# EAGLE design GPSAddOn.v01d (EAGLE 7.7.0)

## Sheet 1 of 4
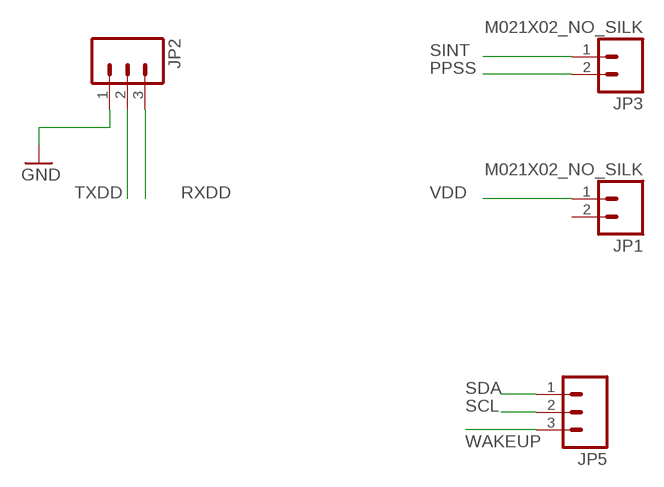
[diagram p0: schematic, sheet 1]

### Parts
JP1  M021X02_NO_SILK  [1X02_NO_SILK]
JP2  M031X03_NO_SILK  [1X03_NO_SILK]
JP3  M021X02_NO_SILK  [1X02_NO_SILK]
JP5  M031X03_NO_SILK  [1X03_NO_SILK]

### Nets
GND: JP2.1 ; also sheet 2,3,4
PPSS: JP3.2 ; also sheet 2
RXDD: JP2.3 ; also sheet 2
SCL: JP5.2 ; also sheet 2,4
SDA: JP5.1 ; also sheet 2,4
SINT: JP3.1 ; also sheet 4
TXDD: JP2.2 ; also sheet 2
VDD: JP1.1 ; also sheet 2,3,4
WAKEUP: JP5.3 ; also sheet 2
Unconnected: JP1.2

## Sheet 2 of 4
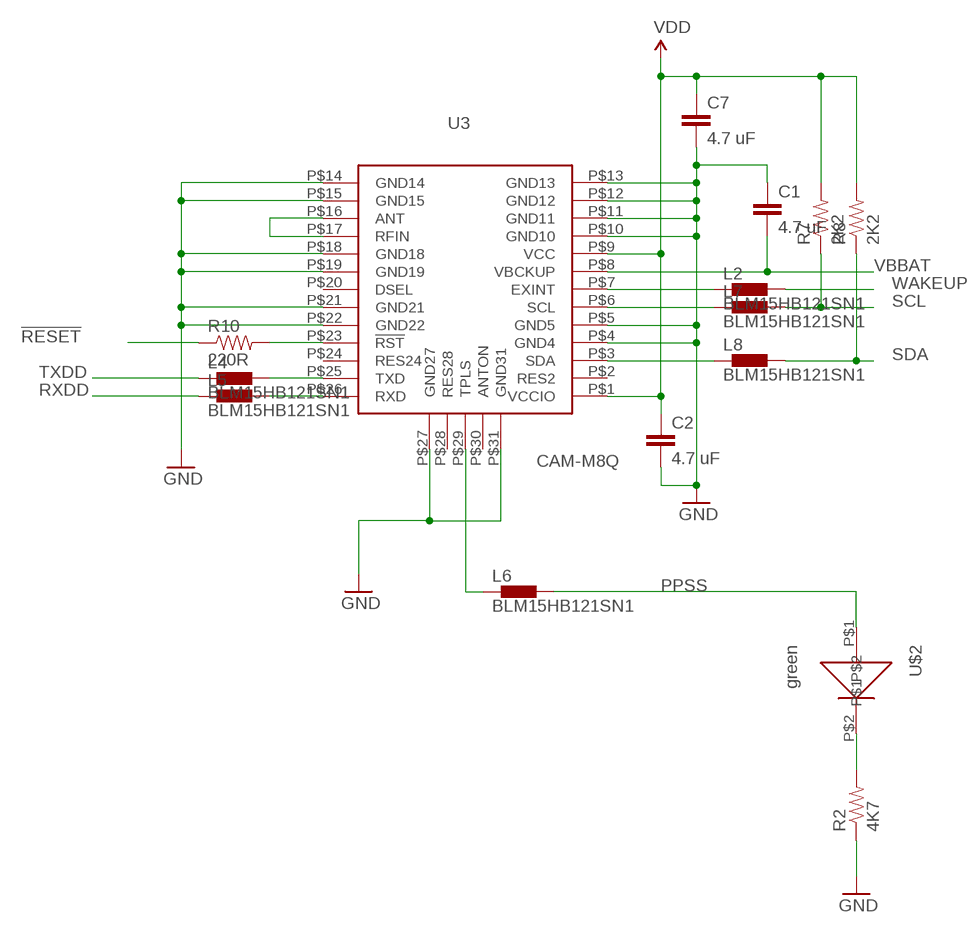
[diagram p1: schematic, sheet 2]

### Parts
C1  4.7 uF  0402CAP.KW  [0402-CAP]
C2  4.7 uF  0402CAP.KW  [0402-CAP]
C7  4.7 uF  0402CAP.KW  [0402-CAP]
L2  BLM15HB121SN1  [0402]
L4  BLM15HB121SN1  [0402]
L5  BLM15HB121SN1  [0402]
L6  BLM15HB121SN1  [0402]
L7  BLM15HB121SN1  [0402]
L8  BLM15HB121SN1  [0402]
R2  4K7  0402RES.KW  [0402-RES]
R7  2K2  0402RES.KW  [0402-RES]
R8  2K2  0402RES.KW  [0402-RES]
R10  220R  0402RES.KW  [0402-RES]
U3  CAM-M8Q  [CAM-M8Q]
U$2  green  0402LED  [0402LED]

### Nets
!RESET: R10.1
GND: C1.1 C2.2 C7.2 R2.1 U3.P$4(GND4) U3.P$5(GND5) U3.P$10(GND10) U3.P$11(GND11) U3.P$12(GND12) U3.P$13(GND13) U3.P$14(GND14) U3.P$15(GND15) U3.P$18(GND18) U3.P$19(GND19) U3.P$21(GND21) U3.P$22(GND22) U3.P$27(GND27) U3.P$31(GND31) ; also sheet 1,3,4
N$6: L2.1 U3.P$7(EXINT)
N$10: L7.1 U3.P$6(SCL)
N$17: R2.2 U$2.P$2
N$23: L8.1 U3.P$3(SDA)
N$43: L4.2 U3.P$25(TXD)
N$44: L5.2 U3.P$26(RXD)
N$45: U3.P$16(ANT) U3.P$17(RFIN)
N$46: R10.2 U3.P$23(!RST)
N$47: L6.1 U3.P$29(TPLS)
PPSS: L6.2 U$2.P$1 ; also sheet 1
RXDD: L5.1 ; also sheet 1
SCL: L7.2 R7.1 ; also sheet 1,4
SDA: L8.2 R8.1 ; also sheet 1,4
TXDD: L4.1 ; also sheet 1
VBBAT: C1.2 U3.P$8(VBCKUP) ; also sheet 3
VDD: C2.1 C7.1 R7.2 R8.2 U3.P$1(VCCIO) U3.P$9(VCC) ; also sheet 1,3,4
WAKEUP: L2.2 ; also sheet 1
Unconnected: U3.P$2(RES2) U3.P$20(DSEL) U3.P$24(RES24) U3.P$28(RES28) U3.P$30(ANTON)

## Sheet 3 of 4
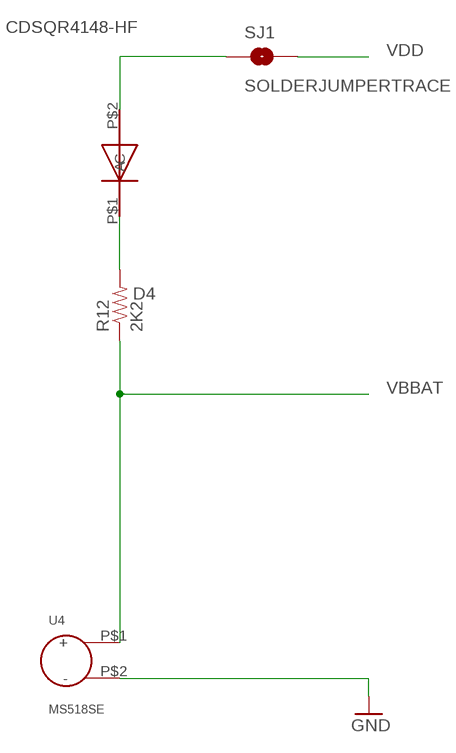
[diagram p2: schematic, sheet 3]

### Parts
D4  CDSQR4148-HF  [CDSQR4148-HF]
R12  2K2  0402RES.KW  [0402-RES]
SJ1  SOLDERJUMPERTRACE  [SJ_2S-TRACE]
U4  MS518SE  [MS518SE]

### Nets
GND: U4.P$2(-) ; also sheet 1,2,4
N$1: D4.P$1(C) R12.2
N$4: D4.P$2(A) SJ1.1
VBBAT: R12.1 U4.P$1(+) ; also sheet 2
VDD: SJ1.2 ; also sheet 1,2,4

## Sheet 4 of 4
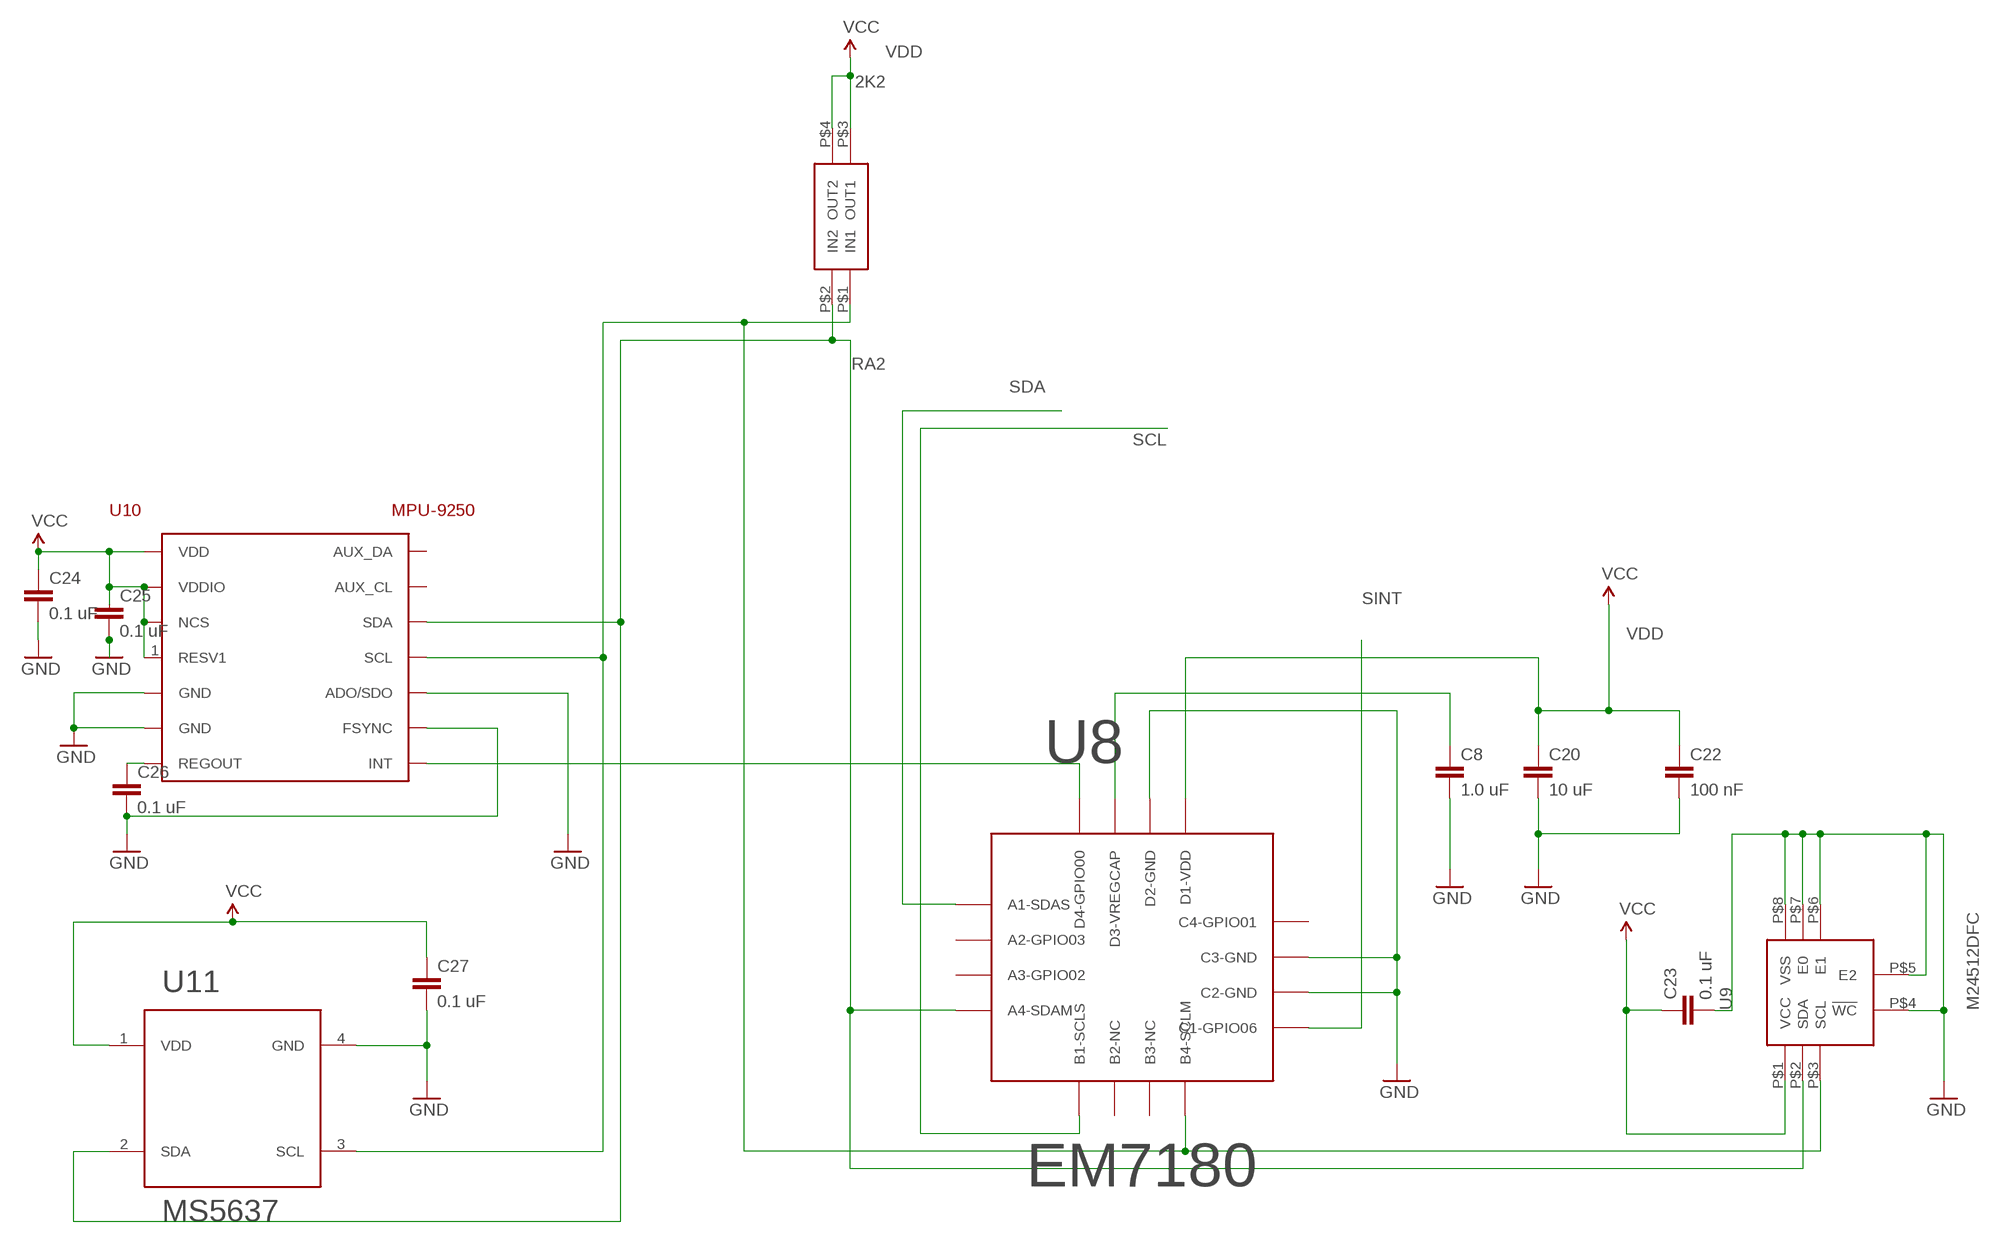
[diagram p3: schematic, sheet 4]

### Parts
C8  1.0 uF  CAP0402-CAP  [0402-CAP]
C20  10 uF  CAP0402-CAP  [0402-CAP]
C22  100 nF  CAP0402-CAP  [0402-CAP]
C23  0.1 uF  CAP0402-CAP  [0402-CAP]
C24  0.1 uF  CAP0402-CAP  [0402-CAP]
C25  0.1 uF  CAP0402-CAP  [0402-CAP]
C26  0.1 uF  CAP0402-CAP  [0402-CAP]
C27  0.1 uF  CAP0402-CAP  [0402-CAP]
RA2  2K2  EXB24V  [EXB24V]
U8  EM7180  [WL-CSP16]
U9  M24512DFC  [M24512DFC]
U10  MPU-9250  [MPU-9250]
U11  MS5637  [MS5637QFN-4]

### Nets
GND: C8.2 C20.2 C22.2 C23.2 C24.2 C25.2 C26.2 C27.2 U8.P$10(C2-GND) U8.P$11(C3-GND) U8.P$14(D2-GND) U9.P$4(!WC) U9.P$5(E2) U9.P$6(E1) U9.P$7(E0) U9.P$8(VSS) U10.9(ADO/SDO) U10.11(FSYNC) U10.18(GND) U10.20(GND) U11.4(GND) ; also sheet 1,2,3
N$19: U8.P$16(D4-GPIO00) U10.12(INT)
N$26: C8.1 U8.P$15(D3-VREGCAP)
N$40: C26.1 U10.10(REGOUT)
SCL: U8.P$5(B1-SCLS) ; also sheet 1,2
SCL2: RA2.P$1(IN1) U8.P$8(B4-SCLM) U9.P$3(SCL) U10.23(SCL) U11.3(SCL)
SDA: U8.P$1(A1-SDAS) ; also sheet 1,2
SDA2: RA2.P$2(IN2) U8.P$4(A4-SDAM) U9.P$2(SDA) U10.24(SDA) U11.2(SDA)
SINT: U8.P$9(C1-GPIO06) ; also sheet 1
VDD: C20.1 C22.1 C23.1 C24.1 C25.1 C27.1 RA2.P$3(OUT1) RA2.P$4(OUT2) U8.P$13(D1-VDD) U9.P$1(VCC) U10.1(RESV1) U10.8(VDDIO) U10.13(VDD) U10.22(NCS) U11.1(VDD) ; supply symbol labelled VCC ; also sheet 1,2,3
Unconnected: U8.P$2(A2-GPIO03) U8.P$3(A3-GPIO02) U8.P$6(B2-NC) U8.P$7(B3-NC) U8.P$12(C4-GPIO01) U10.7(AUX_CL) U10.21(AUX_DA)

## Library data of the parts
C1 C2 C7 = SparkFun-Capacitors:0402CAP.KW
C8 C20 C22-C27 = SparkFun-Capacitors:CAP: Capacitor
D4 = Kris:CDSQR4148-HF: ComChip's CDSQR4148-HF high speed 150 mA Io diode
JP1 JP3 = SparkFun-Connectors:M02: Standard 2-pin 0.1" header. Use with
JP2 JP5 = SparkFun-Connectors:M03: Header 3 Standard 3-pin 0.1" header. Use with straight break away headers (SKU : PRT-00116), right angle break away headers (PRT-00553), swiss pins (PRT-00743), machine pins (PRT-00117), and female headers (PRT-00115). Molex polarized connector foot print use with SKU : PRT-08232 with associated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
L2 L4-L8 = inductors:BLM15H: EMIFIL (R) Chip Ferrite Bead for GHz Noise
R2 R7 R8 R10 R12 = SparkFun-Resistors:0402RES.KW
RA2 = Kris:EXB24V: Panasonic EXB24 22 Ohm series resistor pair
SJ1 = SparkFun-Passives:SOLDERJUMPER: Solder Jumper
U3 = ubloxLib:CAM-M8Q: CAM-M8Q GPS/GNSS Module https://www.u-blox.com/sites/default/files/CAM-M8_HardwareIntegrationManual_%28UBX-14000014%29.pdf
U4 = Kris:MS518SE: S518SE 3 V rechargable Li battery
U8 = SparkFun-DigitalIC:EM7180: WL-CSP19 package for the EM7180 SENtral sensor fusion hub
U9 = Kris:M24512DFC: ST's M24512DFC6 512 Mbit EEPROM
U10 = SparkFun-Sensors:MPU-9250: The MPU-9250 is a 9-axis motion sensor that contains an accelerometer/gyro sensor (MPU-6500) combined with a magnetometer (AK8963).
U11 = SparkFun-DiscreteSemi:MS5637: MS5637 I2C pressure sensor in QFN-4 package by Measurement Specialties
U$2 = Kris:0402LED: 0402led

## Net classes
1 USB: width 0.254 mm, drill 0.33 mm, clearance 0.159 mm
2 Top GND Pour: clearance 0.762 mm to class 1

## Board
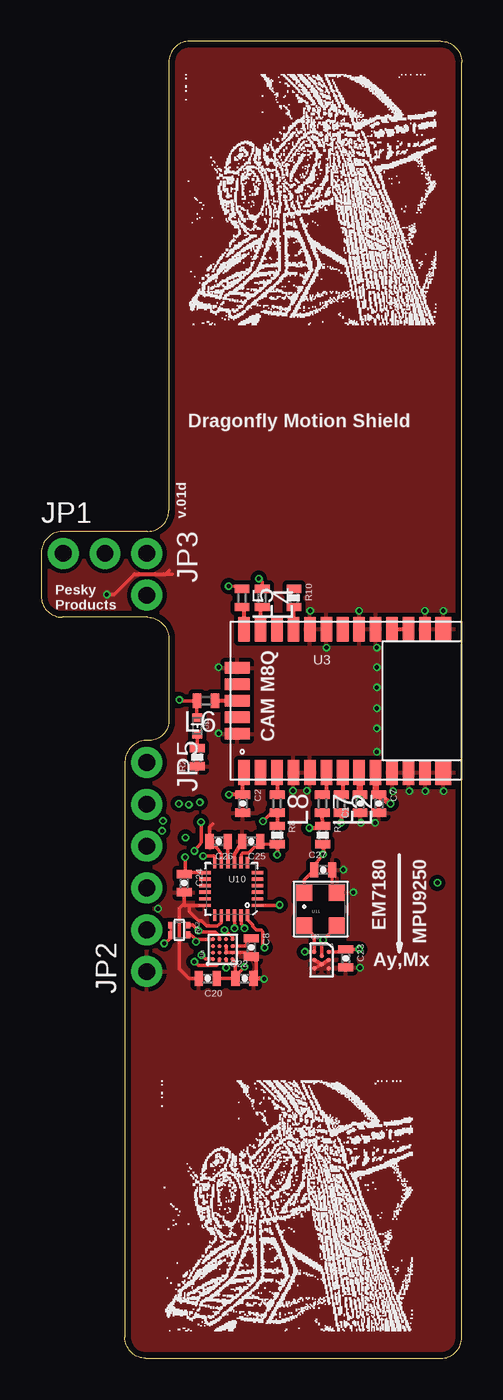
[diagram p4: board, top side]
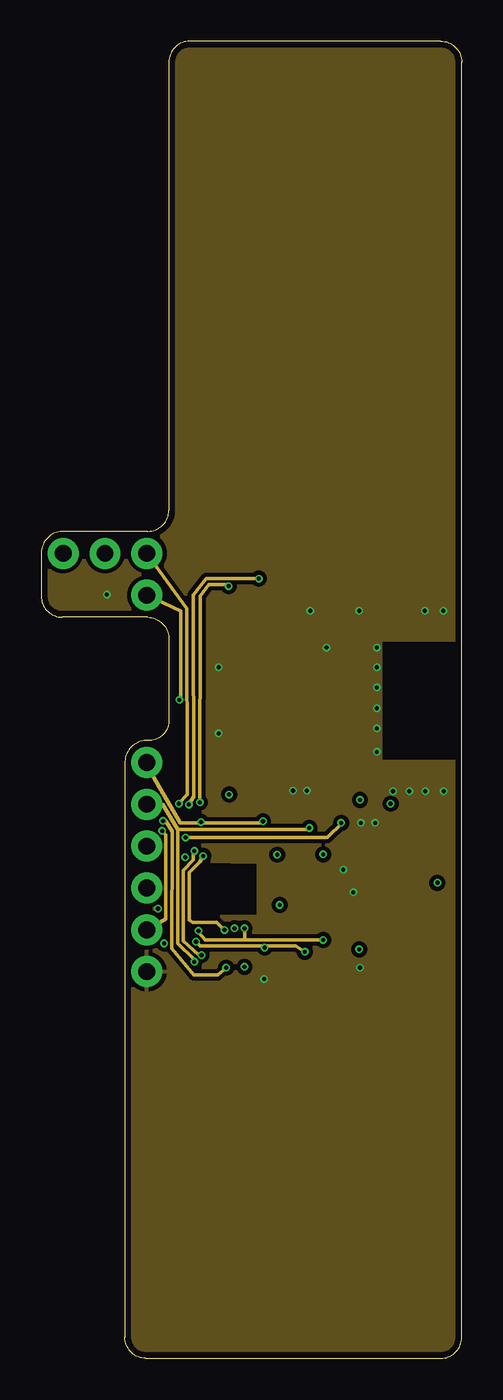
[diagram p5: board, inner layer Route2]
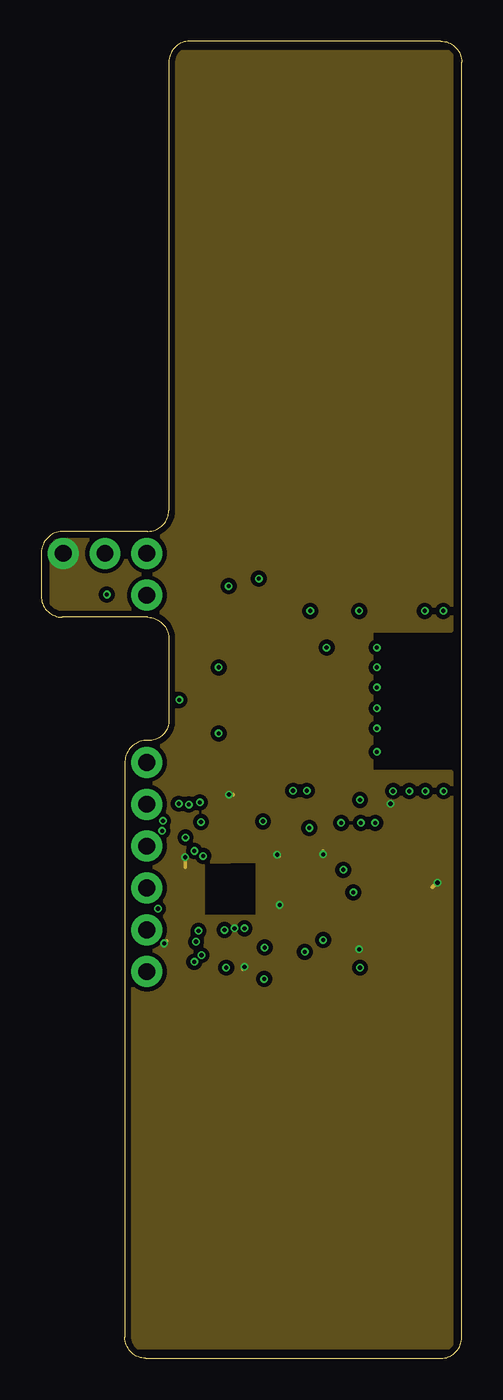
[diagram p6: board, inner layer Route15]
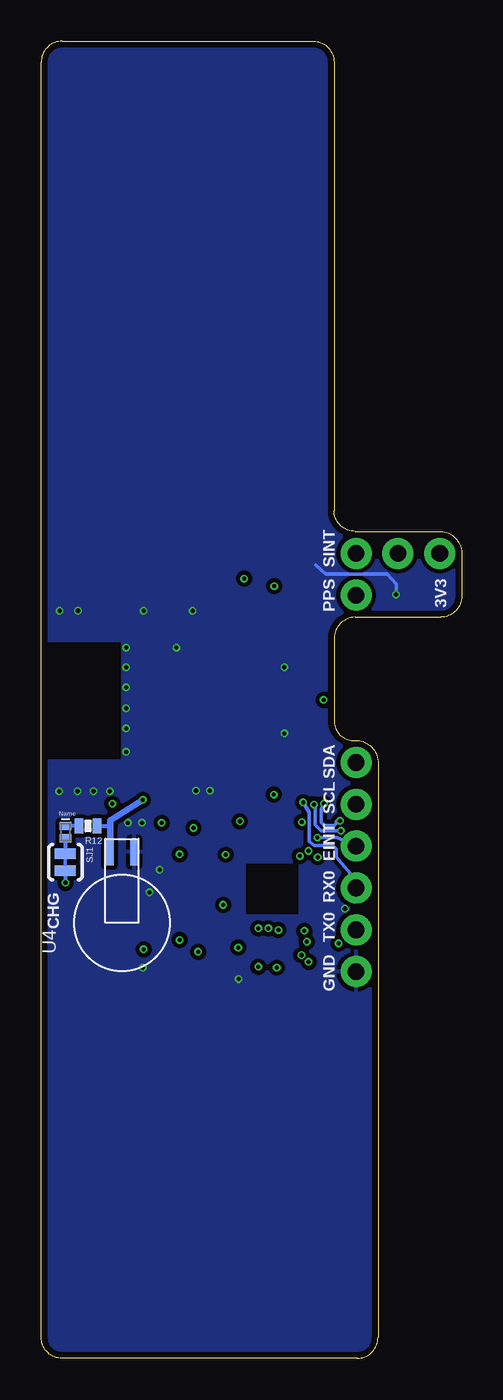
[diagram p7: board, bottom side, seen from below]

Size 25.53 x 79.98 mm. Coordinates in mm from the lower left corner, seen from the top.
Outline: 6.35,0 24.26,0 arc90 25.53,1.27 25.53,78.71 arc90 24.26,79.98 9.02,79.98 arc90 7.75,78.71 7.75,51.49 arc-90 6.48,50.22 1.27,50.22 arc90 0,48.82 0,46.28 arc90 1.27,45.01 6.48,45.01 arc-90 7.75,43.61 7.75,38.66 arc-90 6.48,37.52 arc90 5.08,36.25 5.08,1.27 arc90 6.35,0
Copper layers (1*2*15*16): Top 0.035559375mm / dielectric 0.17018125mm / Route2 0.01778125mm / dielectric 47mil / Route15 0.01778125mm / dielectric 0.17018125mm / Bottom 0.035559375mm
Design rules "OSHPark-4layer *": minimum track width 5mil, minimum drill 10mil, track to track 5mil, track to pad 5mil, pad to pad 5mil, via to via 5mil, smd to smd 5mil, copper to edge 15mil, drill to drill 6mil, minimum pad ring 4mil, minimum via ring 4mil, stop-mask expansion 4mil, vias tented up to drill 20mil, thermal gap 10mil

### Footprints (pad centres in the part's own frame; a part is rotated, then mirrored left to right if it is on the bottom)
0402-CAP = smd 0.5 x 0.9: 1 -0.55,0; 2 0.55,0
CDSQR4148-HF = smd 0.7 x 0.5: P$1 0,0.375; P$2 0,-0.375
1X02_NO_SILK = drill 1.016 pad 1.88: 1 0,0; 2 2.54,0
1X03_NO_SILK = drill 1.016 pad 1.88: 1 0,0; 2 2.54,0; 3 5.08,0
0402 = smd 0.5 x 0.9: 1 -0.55,0; 2 0.55,0
0402-RES = smd 0.5 x 0.9: 1 -0.55,0; 2 0.55,0
EXB24V = smd 0.4 x 0.36: P$1 -0.3,0.5; P$2 0.3,0.5; P$3 -0.3,-0.5; P$4 0.3,-0.5
SJ_2S-TRACE = smd 0.635 x 1.27: 1 -0.508,0; 2 0.508,0
CAM-M8Q = smd 0.7 x 1.5: P$1 0.8,0.45; P$2 1.8,0.45; P$3 2.8,0.45; P$4 3.8,0.45; P$5 4.8,0.45; P$6 5.8,0.45; P$7 6.8,0.45; P$8 7.8,0.45; P$9 8.8,0.45; P$10 9.8,0.45; P$11 10.8,0.45; P$12 11.8,0.45; P$15 11.8,9.15; P$16 10.8,9.15; P$17 9.8,9.15; P$18 8.8,9.15; P$19 7.8,9.15; P$20 6.8,9.15; P$21 5.8,9.15; P$22 4.8,9.15; P$23 3.8,9.15; P$24 2.8,9.15; P$25 1.8,9.15; P$26 0.8,9.15 | smd 1 x 1.5: P$13 12.9,0.45; P$14 12.9,9.15 | smd 1.5 x 0.7: P$27 0.4,6.8; P$28 0.4,5.8; P$29 0.4,4.8; P$30 0.4,3.8; P$31 0.4,2.8
MS518SE = smd 1.6 x 0.5: P$1 4.3,0.75; P$2 4.3,-0.75
WL-CSP16 = smd 0.24 x 0.24: P$1 -0.6,0.6; P$2 -0.2,0.6; P$3 0.2,0.6; P$4 0.6,0.6; P$5 -0.6,0.2; P$6 -0.2,0.2; P$7 0.2,0.2; P$8 0.6,0.2; P$9 -0.6,-0.2; P$10 -0.2,-0.2; P$11 0.2,-0.2; P$12 0.6,-0.2; P$13 -0.6,-0.6; P$14 -0.2,-0.6; P$15 0.2,-0.6; P$16 0.6,-0.6
M24512DFC = smd 0.27 x 0.27: P$1 0.433,0.5; P$2 -0.433,0.5; P$3 0,0.25; P$4 0.433,0; P$5 -0.433,0; P$6 0,-0.25; P$7 0.433,-0.5; P$8 -0.433,-0.5
MPU-9250 = smd 0.7 x 0.2: 1 -1.6,1; 2 -1.6,0.6; 3 -1.6,0.2; 4 -1.6,-0.2; 5 -1.6,-0.6; 6 -1.6,-1; 13 1.6,-1; 14 1.6,-0.6; 15 1.6,-0.2; 16 1.6,0.2; 17 1.6,0.6; 18 1.6,1 | smd 0.2 x 0.7: 7 -1,-1.6; 8 -0.6,-1.6; 9 -0.2,-1.6; 10 0.2,-1.6; 11 0.6,-1.6; 12 1,-1.6; 19 1,1.6; 20 0.6,1.6; 21 0.2,1.6; 22 -0.2,1.6; 23 -0.6,1.6; 24 -1,1.6
MS5637QFN-4 = smd 1 x 1: 1 -1,1; 2 -1,-1; 3 1,-1; 4 1,1
0402LED = smd 0.5 x 0.6: P$1 -0.5,0; P$2 0.5,0

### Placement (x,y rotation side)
C1  19.35,33.68 90 top
C2  12.24,33.68 270 top
C7  20.5,33.68 270 top
C8  12.75,24.94 270 top
C20  10.11,23.06 180 top
C22  12.34,23.06 0 top
C23  18.49,24.28 270 top
C24  8.69,28.85 270 top
C25  12.75,31.39 180 top
C26  10.77,31.39 180 top
C27  17.12,29.67 0 top
D4  24.05,31.95 0 bottom
JP1  1.33,48.88 0 top
JP2  6.41,23.48 90 top
JP3  6.41,48.88 270 top
JP5  6.41,36.18 270 top
L2  18.21,33.68 270 top
L4  13.41,46.18 270 top
L5  12.19,46.18 270 top
L6  10.01,39.93 180 top
L7  17.07,33.68 270 top
L8  14.33,33.68 270 top
R2  9.47,36.5 90 top
R7  17.09,31.78 270 top
R8  14.33,31.78 270 top
R10  15.34,46.18 270 top
R12  22.68,32.33 180 bottom
RA2  8.38,26.01 270 top
SJ1  24.05,30.12 270 bottom
U3  11.51,35.13 0 top
U4  20.62,26.44 90 bottom
U8  11.02,24.84 90 top
U9  17.02,24.18 0 top
U10  11.53,28.5 180 top
U11  16.97,27.28 0 top
U$2  9.47,38.4 270 top

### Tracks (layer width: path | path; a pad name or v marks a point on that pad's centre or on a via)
GND  (via drill 0.25)
  Top 0.152: C27.2 17.67,28.58 U11.4
  Top 0.203: U8.P$11 U8.P$10 U8.P$14 12.5,24.64 C8.2 12.75,24.38 13.06,24.08 13.06,23.22 C22.2 | U10.11 10.93,30.62 10.62,31.04 10.58,31.04 C26.2 10.22,32.27 10.41,32.46 | U10.9 11.73,30.57 C25.2 | 9.91,27.47 U10.18 8.94,27.5 | U9.P$5 U9.P$6 | U9.P$8 U9.P$6 | U9.P$4 U9.P$6 | U10.20 10.93,26.45 10.69,26.26 10.06,26.26 9.75,26.57 9.55,26.57 8.99,27.13 8.99,27.45 8.94,27.5 | 13.26,23.09 12.89,23.09 C22.2 | 7.77,47.83 7.54,47.6 5.66,47.6 4.45,46.38 4.09,46.38 4.06,46.41 3.99,46.41 | C24.2 8.69,27.64 8.62,27.57 | 8.62,27.57 8.38,27.33 8.38,23.65 8.97,23.06 C20.2 | 8.94,27.5 8.7,27.5 8.62,27.57 | 12.9,22.99 12.9,23.05 C22.2 | v13.54,23.04 12.92,23.04 C22.2 | 5.66,47.62 7.95,47.62
  Bottom 0.203: v3.99,46.38 3.99,47.02 4.52,47.62 8.26,47.62 8.87,48.16
  other vias: 23.29,45.39 24.41,45.39 20.37,43.15 19.3,45.39 21.36,34.44 22.35,34.44 23.32,34.44 24.43,34.44 17.32,43.15 16.33,45.39 16.13,34.47 15.29,34.47 10.77,41.96 10.77,37.95 20.37,41.96 20.37,40.74 20.37,39.47 20.37,38.25 20.37,36.83 20.27,32.51 18.95,28.3 18.34,29.67 19.35,23.72 7.09,27.31 19.41,32.51
  pour Top (isolate 0.254): 0,0 0,79.98 25.53,79.98 25.6,43.61 20.57,43.61 20.57,36.25 25.5,36.25 25.5,0 18.54,0 18.54,28.91 15.29,28.91 15.29,25.7 18.49,25.7 18.49,0 13.21,0 13.21,30.18 9.8,30.18 9.8,26.82 13.2,26.82 13.2,0
  pour Route2 (isolate 0.254): 0,0 0,79.98 25.5,79.98 25.58,43.61 20.57,43.61 20.57,36.25 25.58,36.25 25.53,0 13.21,0 13.21,30.12 9.8,30.18 9.8,26.82 13.16,26.82 13.16,0
  pour Bottom (isolate 0.254): 0,0 0,79.98 25.53,79.98 25.53,43.61 20.57,43.61 20.57,36.25 25.53,36.25 25.53,0 13.21,0 13.21,30.18 9.8,30.18 9.8,26.82 13.2,26.82 13.2,0
N$1
  Bottom 0.254: R12.2 D4.P$1
N$4
  Bottom 0.254: D4.P$2 SJ1.1
N$6
  Top 0.254: U3.P$7 18.31,34.25 L2.1
N$10
  Top 0.254: U3.P$6 17.31,34.42 L7.1
N$17
  Top 0.203: U$2.P$2 R2.2
N$19  (via drill 0.25)
  Top 0.203: U8.P$16 11.62,25.56 v11.13,26.01 | v9.83,30.51 10.47,30.51 10.53,30.47 U10.12
  Route2 0.203: v11.13,26.01 10.67,26.47 9.2,26.47 8.99,26.62 8.99,29.51 9.63,30.15 v9.83,30.51
N$23
  Top 0.254: U3.P$3 L8.1
N$26
  Top 0.203: U8.P$15 12.4,25.04 C8.1
N$40
  Top 0.203: U10.10 11.33,31.2 C26.1
N$43
  Top 0.254: U3.P$25 13.33,45.6 13.38,45.6 L4.2
N$44
  Top 0.254: U3.P$26 12.33,45.64 12.32,45.63 L5.2
N$45
  Top 0.254: U3.P$17 U3.P$16
N$46
  Top 0.254: U3.P$23 15.33,45.72 R10.2
N$47
  Top 0.254: U3.P$29 10.79,39.93 L6.1
PPSS  (via drill 0.25)
  Top 0.203: v8.38,39.98 8.44,39.93 L6.2 9.46,39 U$2.P$1
  Route2 0.203: JP3.2 8.48,45.39 8.48,40.13 v8.38,39.98
RXDD  (via drill 0.25)
  Top 0.203: L5.1 11.83,46.88 v11.38,46.89
  Route2 0.203: v9.63,33.76 9.65,46.3 10.19,46.99 11.28,46.99 v11.38,46.89
  Bottom 0.203: JP2.3 6.4,28.57 6.4,28.96 6.76,29.44 7.62,30.45 7.62,30.94 7.82,31.14 8.94,31.14 9.22,31.37 9.25,31.39 9.25,33.15 v9.63,33.76
SCL  (via drill 0.25)
  Top 0.203: U8.P$5 10.82,24.03 10.64,23.85 9.53,23.85 v9.3,24.08
  Top 0.254: v16.28,32.21 16.65,32.21 R7.1 L7.2
  Route2 0.203: 8.28,32.11 16.21,32.11 v16.28,32.21 | v9.3,24.08 9.3,24.23 8.28,25.2 8.28,32.11 | 8.28,32.11 7.37,33.63 6.43,33.63 JP5.2
SCL2  (via drill 0.25)
  Top 0.203: U8.P$8 10.82,25.65 10.57,25.91 9.6,25.91 v9.55,25.96 9.2,26.31 RA2.P$1 | U9.P$3 17.02,25.33 | 17.02,25.33 U11.3 | 17.02,25.33 17.09,25.33 v17.12,25.4 | v12.34,26.11 12.14,26.37 12.14,26.86 U10.23
  Route2 0.203: v17.12,25.4 12.34,25.4 | 12.34,25.4 v12.34,26.11 | v9.55,25.96 9.55,25.86 9.96,25.4 12.34,25.4
SDA  (via drill 0.25)
  Top 0.203: 13.98,33.13 v13.46,32.61 | v9.3,30.81 9.53,31.09 9.7,31.32 v9.7,32.56 | U8.P$1 9.97,24.24 v9.73,24.49
  Top 0.254: R8.1 L8.2 13.98,33.13
  Route2 0.203: v13.46,32.61 13.36,32.51 9.75,32.51 v9.7,32.56 9.65,32.51 8.43,32.51 6.63,35.64 6.63,35.97 JP5.1 | v9.73,24.49 9.58,24.49 8.64,25.35 8.64,29.62 9.25,30.28 9.25,30.61 v9.3,30.81
SDA2  (via drill 0.25)
  Top 0.203: U8.P$4 9.4,25.44 | 15.78,26.11 U11.2 16.59,25.66 U9.P$2 16.58,24.69 v16,24.69 | 9.4,25.44 9.4,25.41 v9.4,25.3 | RA2.P$2 9.09,25.71 9.4,25.44 | U10.24 12.53,26.64 12.85,26.31 12.85,26.21 13.06,26.01 13.36,26.01 13.46,25.91 13.46,25.04 v13.56,24.94
  Route2 0.203: v16,24.69 15.44,25.04 13.56,25.04 | 13.56,25.04 9.65,25.04 v9.4,25.3 | v13.56,24.94 13.56,25.04
SINT  (via drill 0.25)
  Top 0.203: U8.P$9 11.22,23.87 v11.23,23.72
  Route2 0.203: v11.23,23.72 10.72,23.29 9.27,23.29 7.93,24.89 7.95,32 7.57,32.64 v7.39,32.64 | JP3.1 8.84,45.52 8.87,34.24 v8.36,33.68
  Bottom 0.203: v7.39,32.64 7.57,32.64 7.62,32.59 7.62,32.49 7.75,32.36 8.36,32.36 8.53,32.54 8.53,33.38 v8.36,33.68
TXDD  (via drill 0.25)
  Top 0.203: L4.1 13.41,47.14 v13.21,47.35
  Route2 0.203: v13.21,47.35 10.01,47.35 9.25,46.35 9.27,34.11 v8.97,33.63 | v7.34,32.03 7.57,31.78 7.57,26.67 JP2.2
  Bottom 0.203: v7.34,32.03 8.53,32.03 8.89,32.38 8.89,33.55 v8.97,33.63
VBBAT  (via drill 0.25)
  Top 0.406: U3.P$8 19.33,34.33 C1.2 v19.36,33.91
  Bottom 0.254: R12.1 21.38,32.34 21.33,32.38
  Bottom 0.406: v19.36,33.91 21.33,32.67 21.33,32.38 21.33,31.33 21.38,31.28 U4.P$1
VDD  (via drill 0.25)
  Top 0.203: U8.P$13 11.79,23.89 C22.1 | C22.1 11.74,23.12 v12.34,23.77 | U10.22 v11.74,26.11 | U11.1 15.97,29.06 C27.1 16.57,29.93 v17.12,30.61 | v19.3,24.84 19.35,24.83 C23.1 18.59,24.68 U9.P$1 | v7.47,25.2 7.88,25.54 RA2.P$3 RA2.P$4 | R8.2 13.44,31.2 C25.1 12.59,30.68 12.24,30.68 12.13,30.57 U10.8 | v8.74,30.43 8.74,29.57 C24.1 8.71,29.5 U10.13 | U10.1 14.44,27.5 v14.48,27.53 | C20.1 C22.1
  Top 0.254: 20.31,34.45 C7.1 | R7.2 17.13,30.9 v17.12,30.61 | R8.2 v14.33,30.58 | U3.P$1 12.24,35.51 C2.1 11.98,34.23 v11.41,34.24
  Top 0.406: U3.P$9 20.31,34.45 | C7.1 20.67,34.03 v21.21,33.68
  Route15 0.203: v12.34,23.77 12.24,23.62 | v11.74,26.11 11.79,26.11 | v19.3,24.84 19.36,24.79 | v7.47,25.2 7.62,25.35 | v8.74,30.43 8.74,29.82 | v14.48,27.53 14.43,27.48
  Route15 0.254: 21.16,33.71 v21.21,33.68 | v17.12,30.61 17.12,30.78 | v14.33,30.58 14.43,30.48 | v11.41,34.24 11.63,34.24 11.66,34.21 | v24.05,28.88 23.75,28.6
  Bottom 0.254: SJ1.2 v24.05,28.88
  pour Route15 (isolate 0.254, no thermals): 0.64,0.64 0.64,79.35 24.89,79.35 24.89,44.17 20.04,44.17 20.04,35.64 24.89,35.64 24.89,0.64 13.16,0.64 13.16,30.18 9.8,30.12 9.8,26.82 13.11,26.87 13.11,0.64
WAKEUP  (via drill 0.25)
  Top 0.254: L2.2 v18.21,32.51
  Route2 0.203: v18.21,32.51 18.26,32.51 17.37,31.62 v8.76,31.62
  Bottom 0.203: v8.76,31.62 7.6,31.62 JP5.3

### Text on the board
tPlace: Dragonfly Motion Shield | v.01d | Pesky / Products | CAM M8Q | EM7180 | MPU9250 | Ay,Mx
bPlace: SINT | 3V3 | PPS | SDA | SCL | EINT | RX0 | CHG | TX0 | GND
